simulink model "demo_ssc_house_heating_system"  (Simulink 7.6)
settings: Solver=ode15s  SolverMode=SingleTasking  StartTime=0.0  StopTime=3600*50  FixedStep=1  MaxStep=10  RelTol=1e-3
InitFcn:
  | Text=12;
  | %   Simscape Demo "House Heating System"
  | max_temp = 23;    % Maximum temperature
  | min_temp = 18;     % Minimum temperature
  | % Walls
  | % House length = 30 m
  | lenHouse = 30;
  | % House width = 10 m
  | widHouse = 10;
  | % House height = 4 m
  | htHouse = 4;
  | wallArea = 2*lenHouse*htHouse + 2*widHouse*htHouse;
  | LWall = .2;
  | wallVolume = wallArea * LWall;
  | wallDensity = 1920;     % kg/m^3
  | wallMass = wallVolume * wallDensity;
  | c_wall = 835;           % J/kg/K
  | kWall = 0.038;  % Thermal conductivity [W/m/K]
  | % -------------------------------
  | % Windows
  | % Number of windows = 6
  | numWindows = 6;
  | % Height of windows = 1 m
  | htWindows = 1;
  | % Width of windows = 1 m
  | widWindows = 1;
  | windowArea = numWindows*htWindows*widWindows;
  | LWindow = .01;
  | windowVolume = windowArea * LWindow;
  | windowDensity = 2700;       % kg/m^3
  | windowMass = windowVolume * windowDensity;
  | c_window = 840;             % J/kg/K
  | kWindow = 0.78;             % Thermal conductivity [W/m/K]
  | % -------------------------------
  | % Roof
  | % Roof pitch = 40 deg
  | pitRoof = 40/180/pi;
  | roofArea =  2*(1/cos(pitRoof/2))*widHouse*lenHouse + tan(pitRoof)*widHouse;
  | LRoof = 0.2;
  | roofVolume = roofArea * LRoof;
  | roofDensity = 32;           % Glass fiber
  | roofMass = roofVolume * roofDensity;
  | kRoof = 0.038;              % Thermal conductivity [W/m/K]
  | c_roof = 835;               % J/kg/K
  | % -------------------------------
  | % Convective heat gransfer coefficients (W/M^2/K)
  | h_A_W = 24;         % Air-wall
  | h_W_Atm = 34;       % Wall-atmosphere
  | h_A_Wnd = 25;       % Air-window
  | h_Wnd_Atm = 32;     % Window-atmosphere
  | h_A_R = 12;         % Air-roof
  | h_R_Atm = 38;       % Roof-atmosphere
  | % -------------------------------
  | %Air
  | % Density of air at sea level = 1.2250 kg/m^3
  | densAir = 1.2250;
  | % Air mass inside the house
  | M_air = (lenHouse*widHouse*htHouse+tan(pitRoof)*widHouse*lenHouse)*densAir;
  | c_air = 1005.4;         % cp of air at 273 K [J/(kg*K]
  | % -------------------------------
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model workspace: external: MATLAB Code (data not in the file)
libraries: fl_lib x31, nesl_utility x10, simulink x1

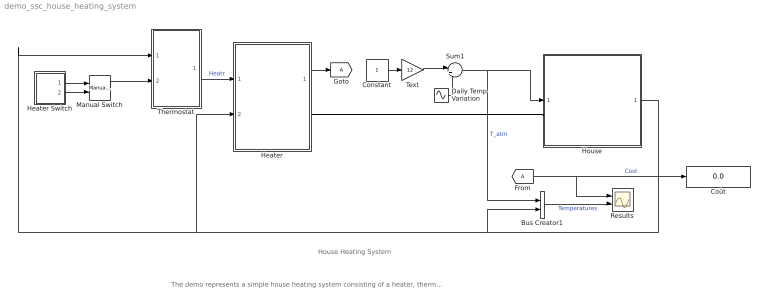
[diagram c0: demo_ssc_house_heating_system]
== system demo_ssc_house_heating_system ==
  note: House Heating System
  note: The demo represents a simple house heating system consisting of a heater, thermostat, and a house structure with four thermally distinguishable parts: inside air, house walls, windows, and roof. The house exchanges heat with the environment through its walls, windows, and roof. Each path is simulated as a combination of a thermal convection, thermal conduction, and the thermal mass. The heater starts pumping hot air if room temperature falls below 18 deg C and is turned off if temperature exceeds 23 deg C. As a result, you can monitor the temperatures of house parts and heat losses through them. The manual switch allows you to investigate system behavior with the heating system turned off.
  Bus Creator1 : BusCreator  Inputs=2
  Constant : Constant
  Coût : Display
  Daily Temp Variation : Sin  Amplitude=8  Frequency=2*pi/(12*3600)  SampleTime=0
  Heater : Subsystem
  Heater Switch : Subsystem
  House : Subsystem
  Manual Switch : simulink/Signal Routing/Manual Switch  SystemSampleTime=-1  sw=1  action=0  varsize=off
  Results : Scope  NumInputPorts=2
  Sum1 : Sum  Inputs=|++
  Text : Gain  Gain=12
  Thermostat : Stateflow chart  TreatAsAtomicUnit=on
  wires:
  Thermostat/1(Heat) -> Heater/1(On/Off)  "Heatr"
  Daily Temp Variation/1 -> Sum1/2
  Text/1 -> Sum1/1
  House/1(Room Temp Troom) -> Bus Creator1/2, Heater/2(Troom), Thermostat/1(Temp)
  Heater/1(HeatCost) -> [A]
  Sum1/1 -> House/1(Outdoor Temp), Bus Creator1/1  "T_atm"
  [A] -> Results/1, Coût/1  "Cost"
  Heater Switch/1(On) -> Manual Switch/1
  Heater Switch/2(Off) -> Manual Switch/2
  Manual Switch/1 -> Thermostat/2(Switch)
  Bus Creator1/1 -> Results/2  "Temperatures"
  Constant/1 -> Text/1
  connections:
  House/LConn1 -- Heater/RConn1

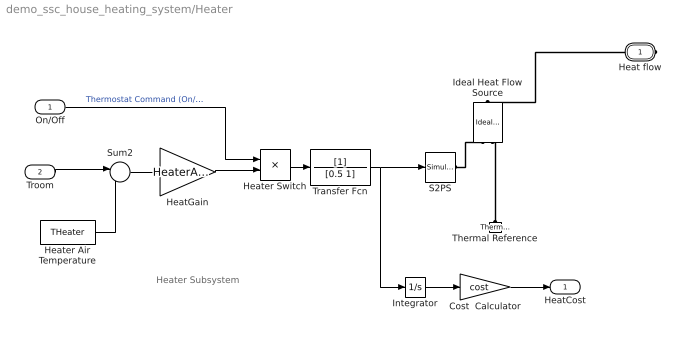
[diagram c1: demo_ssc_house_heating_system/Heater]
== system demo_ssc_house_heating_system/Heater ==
  note: Heater Subsystem
  On/Off : Inport
  Troom : Inport  Port=2
  Cost  Calculator : Gain  Gain=cost
  HeatGain : Gain  Gain=HeaterAirFlow * c_air
  Heater Air Temperature : Constant  Value=THeater
  Heater Switch : Product
  Ideal Heat Flow Source : fl_lib/Thermal/Thermal Sources/Ideal Heat Flow Source  DialogController=NetworkEngine.DynNeDlgSource  SystemSampleTime=-1  Q_Log=off  T_Log=off  LocalVarNames=|heat_flow|T_differential  LocalVarDescs=|Heat flow through the source (J/s)|Temperature differential across the source (K)  LocalVarLogging=[0 0]
  Integrator : Integrator
  S2PS : nesl_utility/Simulink-PS Converter  DialogController=NetworkEngine.DynNeUtilDlgSource  SystemSampleTime=-1  PhysicalDomain=network_engine_domain  LeftPortType=input  RightPortType=output  SubClassName=ps_input  Unit=1  AffineConversion=off  InputFilterTimeConstant=.001  UdotUserProvided=0
  Sum2 : Sum  Inputs=|-+
  Thermal Reference : fl_lib/Thermal/Thermal Elements/Thermal Reference  DialogController=NetworkEngine.DynNeDlgSource  SystemSampleTime=-1  Q_Log=off  LocalVarNames=|Q  LocalVarDescs=|Q  LocalVarLogging=[]
  Transfer Fcn : TransferFcn  Denominator=[0.5 1]
  Heat flow : PMIOPort  Tag=PMCPort  Port=1  Side=Right
  HeatCost : Outport
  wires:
  Heater Air Temperature/1 -> Sum2/2
  Troom/1 -> Sum2/1
  Sum2/1 -> HeatGain/1
  On/Off/1 -> Heater Switch/1  "Thermostat Command (On/Off)"
  HeatGain/1 -> Heater Switch/2
  Heater Switch/1 -> Transfer Fcn/1
  Integrator/1 -> Cost  Calculator/1
  Cost  Calculator/1 -> HeatCost/1
  Transfer Fcn/1 -> S2PS/1, Integrator/1
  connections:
  S2PS/RConn1 -- Ideal Heat Flow Source/RConn1
  Thermal Reference/LConn1 -- Ideal Heat Flow Source/RConn2
  Heat flow/RConn1 -- Ideal Heat Flow Source/LConn1

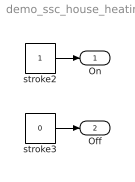
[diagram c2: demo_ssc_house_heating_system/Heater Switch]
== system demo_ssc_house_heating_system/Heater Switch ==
  stroke2 : Constant
  stroke3 : Constant  Value=0
  On : Outport
  Off : Outport  Port=2
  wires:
  stroke2/1 -> On/1
  stroke3/1 -> Off/1

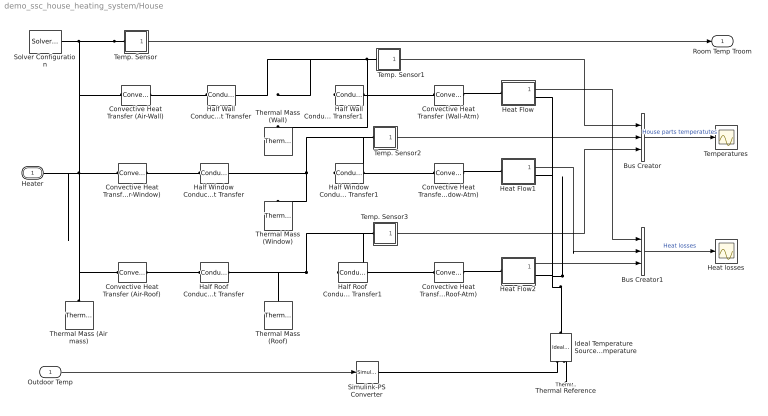
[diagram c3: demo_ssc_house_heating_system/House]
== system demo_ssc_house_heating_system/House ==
  Outdoor Temp : Inport
  Bus Creator : BusCreator  Inputs=3
  Bus Creator1 : BusCreator  Inputs=3
  Convective Heat Transfer (Air-Roof) : fl_lib/Thermal/Thermal Elements/Convective Heat Transfer  DialogController=NetworkEngine.DynNeDlgSource  SystemSampleTime=-1  area=roofArea m^2  heat_tr_coeff=h_A_R W/m^2/K  Q_Log=off  T_Log=off  LocalVarNames=|heat_flow|temperature_diff  LocalVarDescs=|Heat flow (J/s)|Temperature difference (K)  LocalVarLogging=[0 0]
  Convective Heat Transfer (Air-Wall) : fl_lib/Thermal/Thermal Elements/Convective Heat Transfer  DialogController=NetworkEngine.DynNeDlgSource  SystemSampleTime=-1  area=wallArea m^2  heat_tr_coeff=h_A_W W/m^2/K  Q_Log=off  T_Log=off  LocalVarNames=|heat_flow|temperature_diff  LocalVarDescs=|Heat flow (J/s)|Temperature difference (K)  LocalVarLogging=[0 0]
  Convective Heat Transfer (Roof-Atm) : fl_lib/Thermal/Thermal Elements/Convective Heat Transfer  DialogController=NetworkEngine.DynNeDlgSource  SystemSampleTime=-1  area=roofArea m^2  heat_tr_coeff=h_R_Atm W/m^2/K  Q_Log=off  T_Log=off  LocalVarNames=|heat_flow|temperature_diff  LocalVarDescs=|Heat flow (J/s)|Temperature difference (K)  LocalVarLogging=[0 0]
  Convective Heat Transfer (Wall-Atm) : fl_lib/Thermal/Thermal Elements/Convective Heat Transfer  DialogController=NetworkEngine.DynNeDlgSource  SystemSampleTime=-1  area=wallArea m^2  heat_tr_coeff=h_W_Atm W/m^2/K  Q_Log=off  T_Log=off  LocalVarNames=|heat_flow|temperature_diff  LocalVarDescs=|Heat flow (J/s)|Temperature difference (K)  LocalVarLogging=[0 0]
  Convective Heat Transfer (Window-Atm) : fl_lib/Thermal/Thermal Elements/Convective Heat Transfer  DialogController=NetworkEngine.DynNeDlgSource  SystemSampleTime=-1  area=windowArea m^2  heat_tr_coeff=h_Wnd_Atm W/m^2/K  Q_Log=off  T_Log=off  LocalVarNames=|heat_flow|temperature_diff  LocalVarDescs=|Heat flow (J/s)|Temperature difference (K)  LocalVarLogging=[0 0]
  Convective Heat Transfer IAir-Window) : fl_lib/Thermal/Thermal Elements/Convective Heat Transfer  DialogController=NetworkEngine.DynNeDlgSource  SystemSampleTime=-1  area=windowArea m^2  heat_tr_coeff=h_A_Wnd W/m^2/K  Q_Log=off  T_Log=off  LocalVarNames=|heat_flow|temperature_diff  LocalVarDescs=|Heat flow (J/s)|Temperature difference (K)  LocalVarLogging=[0 0]
  Half Roof Conductive Heat Transfer : fl_lib/Thermal/Thermal Elements/Conductive Heat Transfer  DialogController=NetworkEngine.DynNeDlgSource  SystemSampleTime=-1  area=roofArea m^2  thickness=LRoof/2 m  th_cond=kRoof W/m/K  Q_Log=off  T_Log=off  LocalVarNames=|heat_flow|temperature_diff  LocalVarDescs=|Heat flow (J/s)|Temperature difference (K)  LocalVarLogging=[0 0]
  Half Roof Conductive Heat Transfer1 : fl_lib/Thermal/Thermal Elements/Conductive Heat Transfer  DialogController=NetworkEngine.DynNeDlgSource  SystemSampleTime=-1  area=roofArea m^2  thickness=LRoof/2 m  th_cond=kRoof W/m/K  Q_Log=off  T_Log=off  LocalVarNames=|heat_flow|temperature_diff  LocalVarDescs=|Heat flow (J/s)|Temperature difference (K)  LocalVarLogging=[0 0]
  Half Wall Conductive Heat Transfer : fl_lib/Thermal/Thermal Elements/Conductive Heat Transfer  DialogController=NetworkEngine.DynNeDlgSource  SystemSampleTime=-1  area=wallArea m^2  thickness=LWall/2 m  th_cond=kWall W/m/K  Q_Log=off  T_Log=off  LocalVarNames=|heat_flow|temperature_diff  LocalVarDescs=|Heat flow (J/s)|Temperature difference (K)  LocalVarLogging=[0 0]
  Half Wall Conductive Heat Transfer1 : fl_lib/Thermal/Thermal Elements/Conductive Heat Transfer  DialogController=NetworkEngine.DynNeDlgSource  SystemSampleTime=-1  area=wallArea m^2  thickness=LWall/2 m  th_cond=kWall W/m/K  Q_Log=off  T_Log=off  LocalVarNames=|heat_flow|temperature_diff  LocalVarDescs=|Heat flow (J/s)|Temperature difference (K)  LocalVarLogging=[0 0]
  Half Window Conductive Heat Transfer : fl_lib/Thermal/Thermal Elements/Conductive Heat Transfer  DialogController=NetworkEngine.DynNeDlgSource  SystemSampleTime=-1  area=windowArea m^2  thickness=LWindow/2 m  th_cond=kWindow W/m/K  Q_Log=off  T_Log=off  LocalVarNames=|heat_flow|temperature_diff  LocalVarDescs=|Heat flow (J/s)|Temperature difference (K)  LocalVarLogging=[0 0]
  Half Window Conductive Heat Transfer1 : fl_lib/Thermal/Thermal Elements/Conductive Heat Transfer  DialogController=NetworkEngine.DynNeDlgSource  SystemSampleTime=-1  area=windowArea m^2  thickness=LWindow/2 m  th_cond=kWindow W/m/K  Q_Log=off  T_Log=off  LocalVarNames=|heat_flow|temperature_diff  LocalVarDescs=|Heat flow (J/s)|Temperature difference (K)  LocalVarLogging=[0 0]
  Heat Flow : Subsystem
  Heat Flow1 : Subsystem
  Heat Flow2 : Subsystem
  Heat losses : Scope
  Ideal Temperature Source. Outdoor temperature : fl_lib/Thermal/Thermal Sources/Ideal Temperature Source  DialogController=NetworkEngine.DynNeDlgSource  SystemSampleTime=-1  Q_Log=off  T_Log=off  LocalVarNames=|heat_flow|T_differential  LocalVarDescs=|Heat flow rate through the source (J/s)|Temperature differential across the source (K)  LocalVarLogging=[0 0]
  Simulink-PS Converter : nesl_utility/Simulink-PS Converter  DialogController=NetworkEngine.DynNeUtilDlgSource  SystemSampleTime=-1  PhysicalDomain=network_engine_domain  LeftPortType=input  RightPortType=output  SubClassName=ps_input  Unit=C  AffineConversion=on  InputFilterTimeConstant=.001  UdotUserProvided=0
  Solver Configuration : nesl_utility/Solver Configuration  DialogController=NetworkEngine.DynNeUtilDlgSource  SystemSampleTime=-1  PhysicalDomain=network_engine_domain  LeftPortType=input  RightPortType=generic  SubClassName=solver  Accelerate=off  Profile=off  ResidualTolerance=1e-9  MaxNonlinIter=3  MaxModeIter=2  DoFixedCost=off  UseLocalSampling=off  DoDC=off  LinearAlgebra=Sparse  LocalSolverSampleTime=.001  LocalSolverChoice=NE_BACKWARD_EULER_ADVANCER  UseLocalSolver=off
  Temp. Sensor : Subsystem
  Temp. Sensor1 : Subsystem
  Temp. Sensor2 : Subsystem
  Temp. Sensor3 : Subsystem
  Temperatures : Scope
  Thermal Mass (Air mass) : fl_lib/Thermal/Thermal Elements/Thermal Mass  DialogController=NetworkEngine.DynNeDlgSource  SystemSampleTime=-1  mass=M_air kg  sp_heat=c_air J/kg/K  init_temp=TinIC C  Q_Log=off  LocalVarNames=|heat_flow|temperature  LocalVarDescs=|Heat flow (J/s)|Mass temperature (K)  LocalVarLogging=[0 0]
  Thermal Mass (Roof) : fl_lib/Thermal/Thermal Elements/Thermal Mass  DialogController=NetworkEngine.DynNeDlgSource  SystemSampleTime=-1  mass=roofMass kg  sp_heat=c_roof J/kg/K  init_temp=TinIC C  Q_Log=off  LocalVarNames=|heat_flow|temperature  LocalVarDescs=|Heat flow (J/s)|Mass temperature (K)  LocalVarLogging=[0 0]
  Thermal Mass (Wall) : fl_lib/Thermal/Thermal Elements/Thermal Mass  DialogController=NetworkEngine.DynNeDlgSource  SystemSampleTime=-1  mass=wallMass kg  sp_heat=c_wall J/kg/K  init_temp=TinIC C  Q_Log=off  LocalVarNames=|heat_flow|temperature  LocalVarDescs=|Heat flow (J/s)|Mass temperature (K)  LocalVarLogging=[0 0]
  Thermal Mass (Window) : fl_lib/Thermal/Thermal Elements/Thermal Mass  DialogController=NetworkEngine.DynNeDlgSource  SystemSampleTime=-1  mass=windowMass kg  sp_heat=c_window J/kg/K  init_temp=TinIC C  Q_Log=off  LocalVarNames=|heat_flow|temperature  LocalVarDescs=|Heat flow (J/s)|Mass temperature (K)  LocalVarLogging=[0 0]
  Thermal Reference : fl_lib/Thermal/Thermal Elements/Thermal Reference  DialogController=NetworkEngine.DynNeDlgSource  SystemSampleTime=-1  Q_Log=off  LocalVarNames=|Q  LocalVarDescs=|Q  LocalVarLogging=[]
  Heater : PMIOPort  Tag=PMCPort  Port=1  Side=Left
  Room Temp Troom : Outport  InitialOutput=0
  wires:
  Outdoor Temp/1 -> Simulink-PS Converter/1
  Temp. Sensor/1(T) -> Room Temp Troom/1
  Temp. Sensor1/1(T) -> Bus Creator/1
  Temp. Sensor2/1(T) -> Bus Creator/2
  Temp. Sensor3/1(T) -> Bus Creator/3
  Bus Creator/1 -> Temperatures/1  "House parts temperatutes"
  Heat Flow2/1(Q) -> Bus Creator1/3
  Heat Flow1/1(Q) -> Bus Creator1/2
  Heat Flow/1(Q) -> Bus Creator1/1
  Bus Creator1/1 -> Heat losses/1  "Heat losses"
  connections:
  Thermal Reference/LConn1 -- Ideal Temperature Source. Outdoor temperature/RConn2
  Ideal Temperature Source. Outdoor temperature/RConn1 -- Simulink-PS Converter/RConn1
  Temp. Sensor/LConn1 -- Solver Configuration/RConn1 -- Heater/RConn1 -- Thermal Mass (Air mass)/LConn1 -- Convective Heat Transfer (Air-Roof)/LConn1 -- Convective Heat Transfer IAir-Window)/LConn1 -- Convective Heat Transfer (Air-Wall)/LConn1
  Convective Heat Transfer (Air-Wall)/RConn1 -- Half Wall Conductive Heat Transfer/LConn1
  Temp. Sensor1/LConn1 -- Half Wall Conductive Heat Transfer/RConn1 -- Thermal Mass (Wall)/LConn1 -- Half Wall Conductive Heat Transfer1/LConn1
  Half Wall Conductive Heat Transfer1/RConn1 -- Convective Heat Transfer (Wall-Atm)/LConn1
  Convective Heat Transfer IAir-Window)/RConn1 -- Half Window Conductive Heat Transfer/LConn1
  Temp. Sensor2/LConn1 -- Half Window Conductive Heat Transfer/RConn1 -- Thermal Mass (Window)/LConn1 -- Half Window Conductive Heat Transfer1/LConn1
  Half Window Conductive Heat Transfer1/RConn1 -- Convective Heat Transfer (Window-Atm)/LConn1
  Convective Heat Transfer (Air-Roof)/RConn1 -- Half Roof Conductive Heat Transfer/LConn1
  Temp. Sensor3/LConn1 -- Thermal Mass (Roof)/LConn1 -- Half Roof Conductive Heat Transfer/RConn1 -- Half Roof Conductive Heat Transfer1/LConn1
  Half Roof Conductive Heat Transfer1/RConn1 -- Convective Heat Transfer (Roof-Atm)/LConn1
  Convective Heat Transfer (Wall-Atm)/RConn1 -- Heat Flow/LConn1
  Convective Heat Transfer (Window-Atm)/RConn1 -- Heat Flow1/LConn1
  Convective Heat Transfer (Roof-Atm)/RConn1 -- Heat Flow2/LConn1
  Ideal Temperature Source. Outdoor temperature/LConn1 -- Heat Flow/RConn1 -- Heat Flow1/RConn1 -- Heat Flow2/RConn1

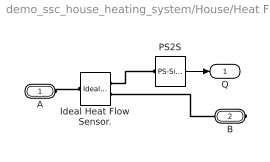
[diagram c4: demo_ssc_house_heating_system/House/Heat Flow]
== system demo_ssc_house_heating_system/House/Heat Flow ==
  Ideal Heat Flow Sensor. : fl_lib/Thermal/Thermal Sensors/Ideal Heat Flow Sensor  DialogController=NetworkEngine.DynNeDlgSource  SystemSampleTime=-1  Q_Log=off  T_Log=off  LocalVarNames=|Q|T  LocalVarDescs=|Q|T  LocalVarLogging=[]
  PS2S : nesl_utility/PS-Simulink Converter  DialogController=NetworkEngine.DynNeUtilDlgSource  SystemSampleTime=-1  PhysicalDomain=network_engine_domain  LeftPortType=input  RightPortType=output  SubClassName=ps_output  Unit=1  AffineConversion=off
  A : PMIOPort  Port=1  Side=Left
  B : PMIOPort  Port=2  Side=Right
  Q : Outport
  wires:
  PS2S/1 -> Q/1
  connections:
  Ideal Heat Flow Sensor./RConn1 -- PS2S/LConn1
  A/RConn1 -- Ideal Heat Flow Sensor./LConn1
  B/RConn1 -- Ideal Heat Flow Sensor./RConn2

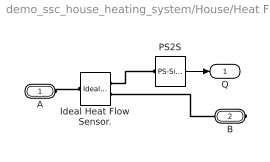
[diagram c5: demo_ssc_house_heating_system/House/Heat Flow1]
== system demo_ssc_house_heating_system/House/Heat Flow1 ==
  Ideal Heat Flow Sensor. : fl_lib/Thermal/Thermal Sensors/Ideal Heat Flow Sensor  DialogController=NetworkEngine.DynNeDlgSource  SystemSampleTime=-1  Q_Log=off  T_Log=off  LocalVarNames=|Q|T  LocalVarDescs=|Q|T  LocalVarLogging=[]
  PS2S : nesl_utility/PS-Simulink Converter  DialogController=NetworkEngine.DynNeUtilDlgSource  SystemSampleTime=-1  PhysicalDomain=network_engine_domain  LeftPortType=input  RightPortType=output  SubClassName=ps_output  Unit=1  AffineConversion=off
  A : PMIOPort  Port=1  Side=Left
  B : PMIOPort  Port=2  Side=Right
  Q : Outport
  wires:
  PS2S/1 -> Q/1
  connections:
  B/RConn1 -- Ideal Heat Flow Sensor./RConn2
  A/RConn1 -- Ideal Heat Flow Sensor./LConn1
  Ideal Heat Flow Sensor./RConn1 -- PS2S/LConn1

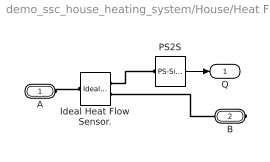
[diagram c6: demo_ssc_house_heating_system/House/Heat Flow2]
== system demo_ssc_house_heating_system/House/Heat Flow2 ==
  Ideal Heat Flow Sensor. : fl_lib/Thermal/Thermal Sensors/Ideal Heat Flow Sensor  DialogController=NetworkEngine.DynNeDlgSource  SystemSampleTime=-1  Q_Log=off  T_Log=off  LocalVarNames=|Q|T  LocalVarDescs=|Q|T  LocalVarLogging=[]
  PS2S : nesl_utility/PS-Simulink Converter  DialogController=NetworkEngine.DynNeUtilDlgSource  SystemSampleTime=-1  PhysicalDomain=network_engine_domain  LeftPortType=input  RightPortType=output  SubClassName=ps_output  Unit=1  AffineConversion=off
  A : PMIOPort  Port=1  Side=Left
  B : PMIOPort  Port=2  Side=Right
  Q : Outport
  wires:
  PS2S/1 -> Q/1
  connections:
  Ideal Heat Flow Sensor./RConn1 -- PS2S/LConn1
  A/RConn1 -- Ideal Heat Flow Sensor./LConn1
  B/RConn1 -- Ideal Heat Flow Sensor./RConn2

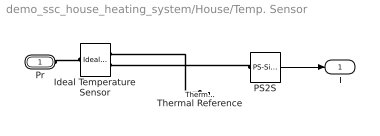
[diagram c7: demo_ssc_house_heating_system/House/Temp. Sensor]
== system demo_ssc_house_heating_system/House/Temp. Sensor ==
  Ideal Temperature Sensor : fl_lib/Thermal/Thermal Sensors/Ideal Temperature Sensor  DialogController=NetworkEngine.DynNeDlgSource  SystemSampleTime=-1  Qs_Log=off  Ts_Log=off  LocalVarNames=|Qs|Ts  LocalVarDescs=|Qs|Ts  LocalVarLogging=[]
  PS2S : nesl_utility/PS-Simulink Converter  DialogController=NetworkEngine.DynNeUtilDlgSource  SystemSampleTime=-1  PhysicalDomain=network_engine_domain  LeftPortType=input  RightPortType=output  SubClassName=ps_output  Unit=C  AffineConversion=on
  Thermal Reference : fl_lib/Thermal/Thermal Elements/Thermal Reference  DialogController=NetworkEngine.DynNeDlgSource  SystemSampleTime=-1  Q_Log=off  LocalVarNames=|Q  LocalVarDescs=|Q  LocalVarLogging=[]
  Pr : PMIOPort  Port=1  Side=Left
  T : Outport
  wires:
  PS2S/1 -> T/1
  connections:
  Ideal Temperature Sensor/RConn1 -- Thermal Reference/LConn1
  PS2S/LConn1 -- Ideal Temperature Sensor/RConn2
  Pr/RConn1 -- Ideal Temperature Sensor/LConn1

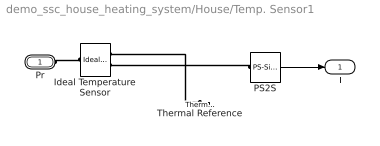
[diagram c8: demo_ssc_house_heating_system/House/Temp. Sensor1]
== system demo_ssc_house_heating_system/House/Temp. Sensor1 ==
  Ideal Temperature Sensor : fl_lib/Thermal/Thermal Sensors/Ideal Temperature Sensor  DialogController=NetworkEngine.DynNeDlgSource  SystemSampleTime=-1  Qs_Log=off  Ts_Log=off  LocalVarNames=|Qs|Ts  LocalVarDescs=|Qs|Ts  LocalVarLogging=[]
  PS2S : nesl_utility/PS-Simulink Converter  DialogController=NetworkEngine.DynNeUtilDlgSource  SystemSampleTime=-1  PhysicalDomain=network_engine_domain  LeftPortType=input  RightPortType=output  SubClassName=ps_output  Unit=C  AffineConversion=on
  Thermal Reference : fl_lib/Thermal/Thermal Elements/Thermal Reference  DialogController=NetworkEngine.DynNeDlgSource  SystemSampleTime=-1  Q_Log=off  LocalVarNames=|Q  LocalVarDescs=|Q  LocalVarLogging=[]
  Pr : PMIOPort  Port=1  Side=Left
  T : Outport
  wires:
  PS2S/1 -> T/1
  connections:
  Pr/RConn1 -- Ideal Temperature Sensor/LConn1
  PS2S/LConn1 -- Ideal Temperature Sensor/RConn2
  Ideal Temperature Sensor/RConn1 -- Thermal Reference/LConn1

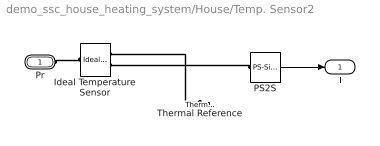
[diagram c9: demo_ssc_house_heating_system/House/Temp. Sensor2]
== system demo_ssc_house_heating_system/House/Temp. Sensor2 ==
  Ideal Temperature Sensor : fl_lib/Thermal/Thermal Sensors/Ideal Temperature Sensor  DialogController=NetworkEngine.DynNeDlgSource  SystemSampleTime=-1  Qs_Log=off  Ts_Log=off  LocalVarNames=|Qs|Ts  LocalVarDescs=|Qs|Ts  LocalVarLogging=[]
  PS2S : nesl_utility/PS-Simulink Converter  DialogController=NetworkEngine.DynNeUtilDlgSource  SystemSampleTime=-1  PhysicalDomain=network_engine_domain  LeftPortType=input  RightPortType=output  SubClassName=ps_output  Unit=C  AffineConversion=on
  Thermal Reference : fl_lib/Thermal/Thermal Elements/Thermal Reference  DialogController=NetworkEngine.DynNeDlgSource  SystemSampleTime=-1  Q_Log=off  LocalVarNames=|Q  LocalVarDescs=|Q  LocalVarLogging=[]
  Pr : PMIOPort  Port=1  Side=Left
  T : Outport
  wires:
  PS2S/1 -> T/1
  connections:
  Ideal Temperature Sensor/RConn1 -- Thermal Reference/LConn1
  PS2S/LConn1 -- Ideal Temperature Sensor/RConn2
  Pr/RConn1 -- Ideal Temperature Sensor/LConn1

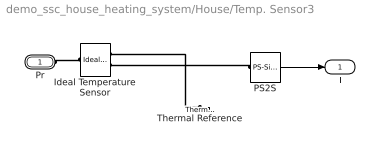
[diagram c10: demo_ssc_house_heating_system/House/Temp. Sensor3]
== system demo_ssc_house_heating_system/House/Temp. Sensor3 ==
  Ideal Temperature Sensor : fl_lib/Thermal/Thermal Sensors/Ideal Temperature Sensor  DialogController=NetworkEngine.DynNeDlgSource  SystemSampleTime=-1  Qs_Log=off  Ts_Log=off  LocalVarNames=|Qs|Ts  LocalVarDescs=|Qs|Ts  LocalVarLogging=[]
  PS2S : nesl_utility/PS-Simulink Converter  DialogController=NetworkEngine.DynNeUtilDlgSource  SystemSampleTime=-1  PhysicalDomain=network_engine_domain  LeftPortType=input  RightPortType=output  SubClassName=ps_output  Unit=C  AffineConversion=on
  Thermal Reference : fl_lib/Thermal/Thermal Elements/Thermal Reference  DialogController=NetworkEngine.DynNeDlgSource  SystemSampleTime=-1  Q_Log=off  LocalVarNames=|Q  LocalVarDescs=|Q  LocalVarLogging=[]
  Pr : PMIOPort  Port=1  Side=Left
  T : Outport
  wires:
  PS2S/1 -> T/1
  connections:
  Pr/RConn1 -- Ideal Temperature Sensor/LConn1
  PS2S/LConn1 -- Ideal Temperature Sensor/RConn2
  Ideal Temperature Sensor/RConn1 -- Thermal Reference/LConn1

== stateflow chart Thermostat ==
  state Heater_on
    entry: Heat =1;
  state Heater_off
    entry: Heat = 0;
  (default) -> Heater_off
  Heater_on -> Heater_off : [(Temp  >max_temp && Switch) | ~Switch]
  Heater_off -> Heater_on : [Temp < min_temp && Switch]
